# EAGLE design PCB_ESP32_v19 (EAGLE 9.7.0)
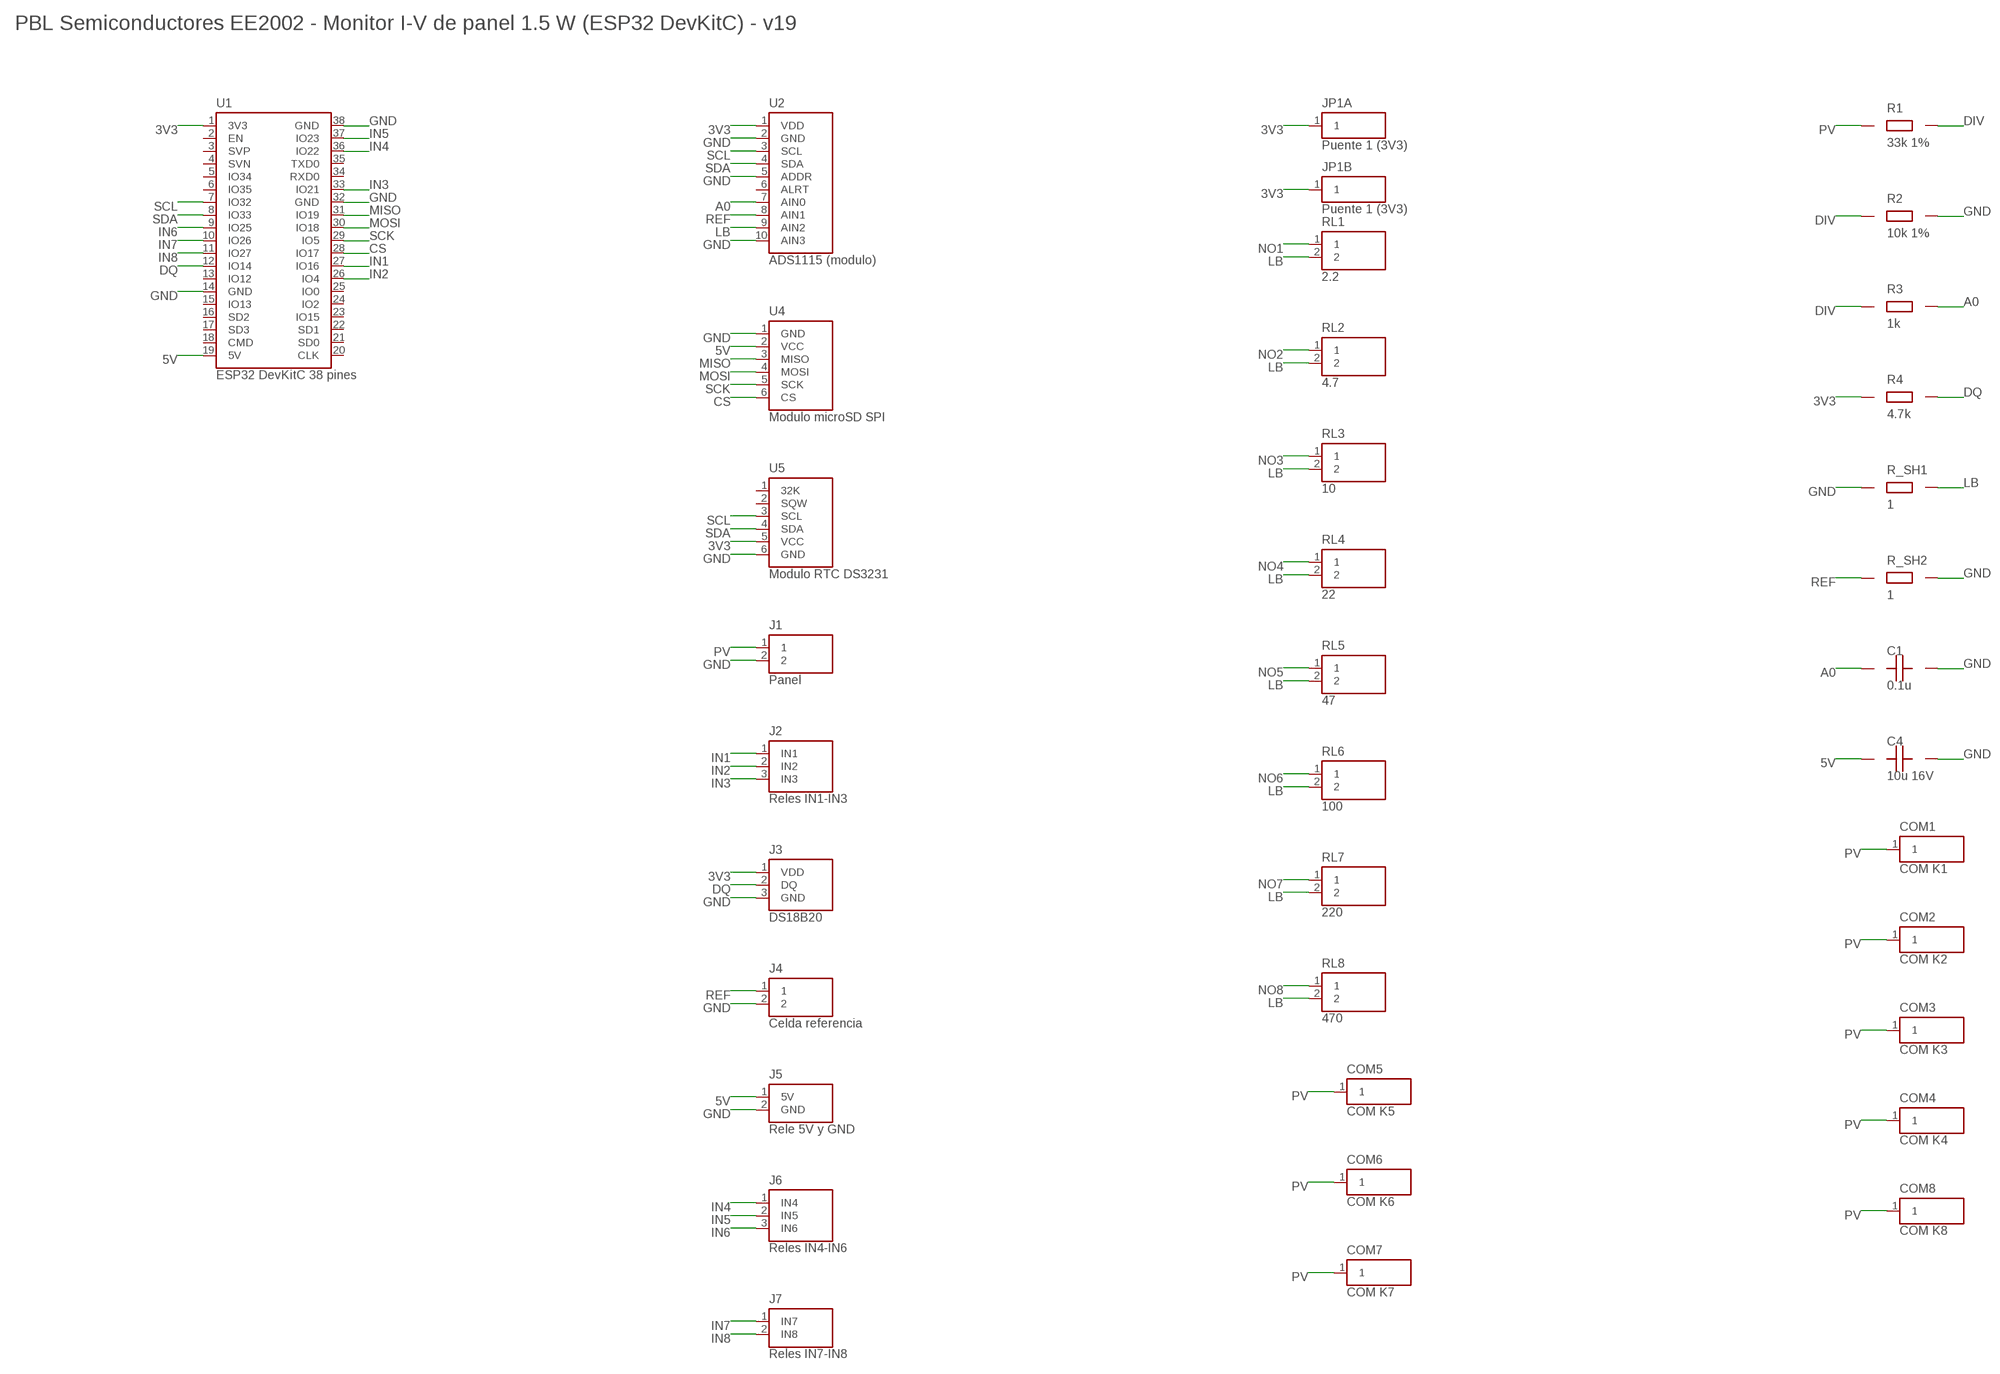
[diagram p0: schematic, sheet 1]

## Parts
C1  0.1u  C  [CAP_5MM]
C4  10u 16V  CP  [CAP_E_2_54]
COM1  COM K1  WIREPAD  [WIREPAD]
COM2  COM K2  WIREPAD  [WIREPAD]
COM3  COM K3  WIREPAD  [WIREPAD]
COM4  COM K4  WIREPAD  [WIREPAD]
COM5  COM K5  WIREPAD  [WIREPAD]
COM6  COM K6  WIREPAD  [WIREPAD]
COM7  COM K7  WIREPAD  [WIREPAD]
COM8  COM K8  WIREPAD  [WIREPAD]
J1  Panel  TERM2  [TERM2_5MM]
J2  Reles IN1-IN3  RELAY_L  [MALE_1X03]
J3  DS18B20  DS18B20_HDR  [MALE_1X03]
J4  Celda referencia  TERM2  [TERM2_5MM]
J5  Rele 5V y GND  RELAY_PWR  [MALE_1X02]
J6  Reles IN4-IN6  RELAY_RA  [MALE_1X03]
J7  Reles IN7-IN8  RELAY_RC  [MALE_1X02]
JP1A  Puente 1 (3V3)  JPAD  [JPAD]
JP1B  Puente 1 (3V3)  JPAD  [JPAD]
R1  33k 1%  R  [RES_V]
R2  10k 1%  R  [RES_V]
R3  1k  R  [RES_V]
R4  4.7k  R  [RES_V]
R_SH1  1  R  [RES_V]
R_SH2  1  R  [RES_V]
RL1  2.2  RLOAD  [RES_H_T]
RL2  4.7  RLOAD  [RES_H_T]
RL3  10  RLOAD  [RES_H_T]
RL4  22  RLOAD  [RES_H_T]
RL5  47  RLOAD  [RES_H_T]
RL6  100  RLOAD  [RES_H_T]
RL7  220  RLOAD  [RES_H_T]
RL8  470  RLOAD  [RES_H_T]
U1  ESP32 DevKitC 38 pines  ESP32  [ESP32_DEVKIT38]
U2  ADS1115 (modulo)  ADS1115  [SOCKET_1X10]
U4  Modulo microSD SPI  SDCARD  [SOCKET_1X06]
U5  Modulo RTC DS3231  DS3231  [SOCKET_1X06]

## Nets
3V3 [POWER]: J3.1(VDD) JP1A.1 JP1B.1 R4.1 U1.1(3V3) U2.1(VDD) U5.5(VCC)
5V [POWER]: C4.1(+) J5.1(5V) U1.19(5V) U4.2(VCC)
A0: C1.1 R3.2 U2.7(AIN0)
CS: U1.28(IO17) U4.6(CS)
DIV: R1.2 R2.1 R3.1
DQ: J3.2(DQ) R4.2 U1.12(IO14)
GND [POWER]: C1.2 C4.2(-) J1.2 J3.3(GND) J4.2 J5.2(GND) R2.2 R_SH1.1 R_SH2.2 U1.14(GND) U1.32(GND) U1.38(GND) U2.2(GND) U2.5(ADDR) U2.10(AIN3) U4.1(GND) U5.6(GND)
IN1: J2.1(IN1) U1.27(IO16)
IN2: J2.2(IN2) U1.26(IO4)
IN3: J2.3(IN3) U1.33(IO21)
IN4: J6.1(IN4) U1.36(IO22)
IN5: J6.2(IN5) U1.37(IO23)
IN6: J6.3(IN6) U1.9(IO25)
IN7: J7.1(IN7) U1.10(IO26)
IN8: J7.2(IN8) U1.11(IO27)
LB [POWER]: R_SH1.2 RL1.2 RL2.2 RL3.2 RL4.2 RL5.2 RL6.2 RL7.2 RL8.2 U2.9(AIN2)
MISO: U1.31(IO19) U4.3(MISO)
MOSI: U1.30(IO18) U4.4(MOSI)
NO1: RL1.1
NO2: RL2.1
NO3: RL3.1
NO4: RL4.1
NO5: RL5.1
NO6: RL6.1
NO7: RL7.1
NO8: RL8.1
PV [POWER]: COM1.1 COM2.1 COM3.1 COM4.1 COM5.1 COM6.1 COM7.1 COM8.1 J1.1 R1.1
REF: J4.1 R_SH2.1 U2.8(AIN1)
SCK: U1.29(IO5) U4.5(SCK)
SCL: U1.7(IO32) U2.3(SCL) U5.3(SCL)
SDA: U1.8(IO33) U2.4(SDA) U5.4(SDA)
Unconnected: U1.2(EN) U1.3(SVP) U1.4(SVN) U1.5(IO34) U1.6(IO35) U1.13(IO12) U1.15(IO13) U1.16(SD2) U1.17(SD3) U1.18(CMD) U1.20(CLK) U1.21(SD0) U1.22(SD1) U1.23(IO15) U1.24(IO2) U1.25(IO0) U1.34(RXD0) U1.35(TXD0) U2.6(ALRT) U5.1(32K) U5.2(SQW)

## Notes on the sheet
- PBL Semiconductores EE2002 - Monitor I-V de panel 1.5 W (ESP32 DevKitC) - v19

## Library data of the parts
C1 = PCB_PBL_Semiconductores:C
C4 = PCB_PBL_Semiconductores:CP
COM1-COM8 = PCB_PBL_Semiconductores:WIREPAD
J1 J4 = PCB_PBL_Semiconductores:TERM2
J2 = PCB_PBL_Semiconductores:RELAY_L
J3 = PCB_PBL_Semiconductores:DS18B20_HDR
J5 = PCB_PBL_Semiconductores:RELAY_PWR
J6 = PCB_PBL_Semiconductores:RELAY_RA
J7 = PCB_PBL_Semiconductores:RELAY_RC
JP1A JP1B = PCB_PBL_Semiconductores:JPAD
R1-R4 R_SH1 R_SH2 = PCB_PBL_Semiconductores:R
RL1-RL8 = PCB_PBL_Semiconductores:RLOAD
U1 = PCB_PBL_Semiconductores:ESP32
U2 = PCB_PBL_Semiconductores:ADS1115
U4 = PCB_PBL_Semiconductores:SDCARD
U5 = PCB_PBL_Semiconductores:DS3231

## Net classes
0 SIGNAL: width 0.254 mm, drill 0.381 mm, clearance 0.254 mm
1 POWER: width 0.381 mm, drill 0.508 mm, clearance 0.305 mm to class 0, clearance 0.305 mm

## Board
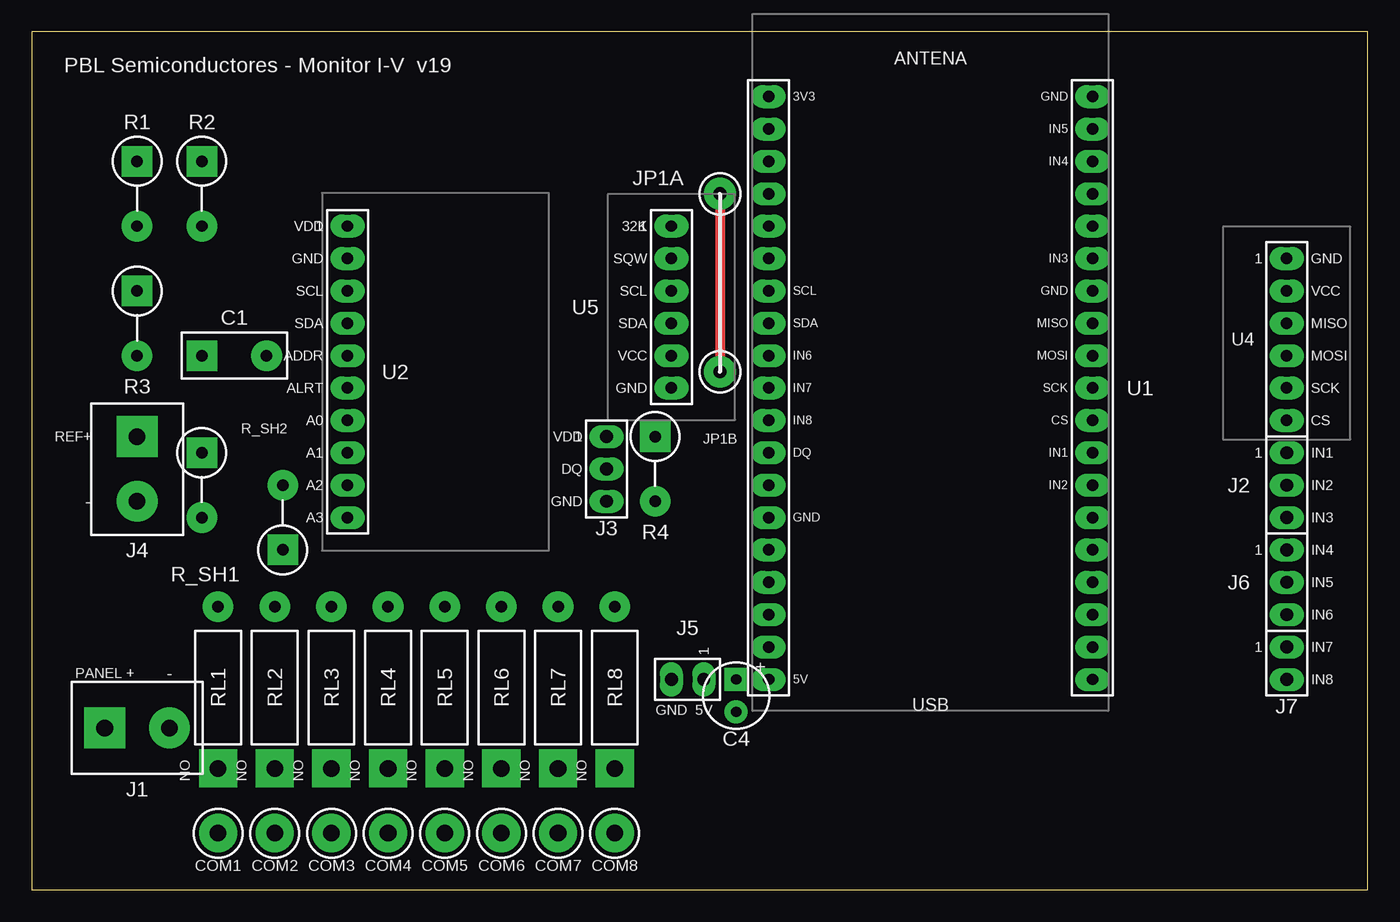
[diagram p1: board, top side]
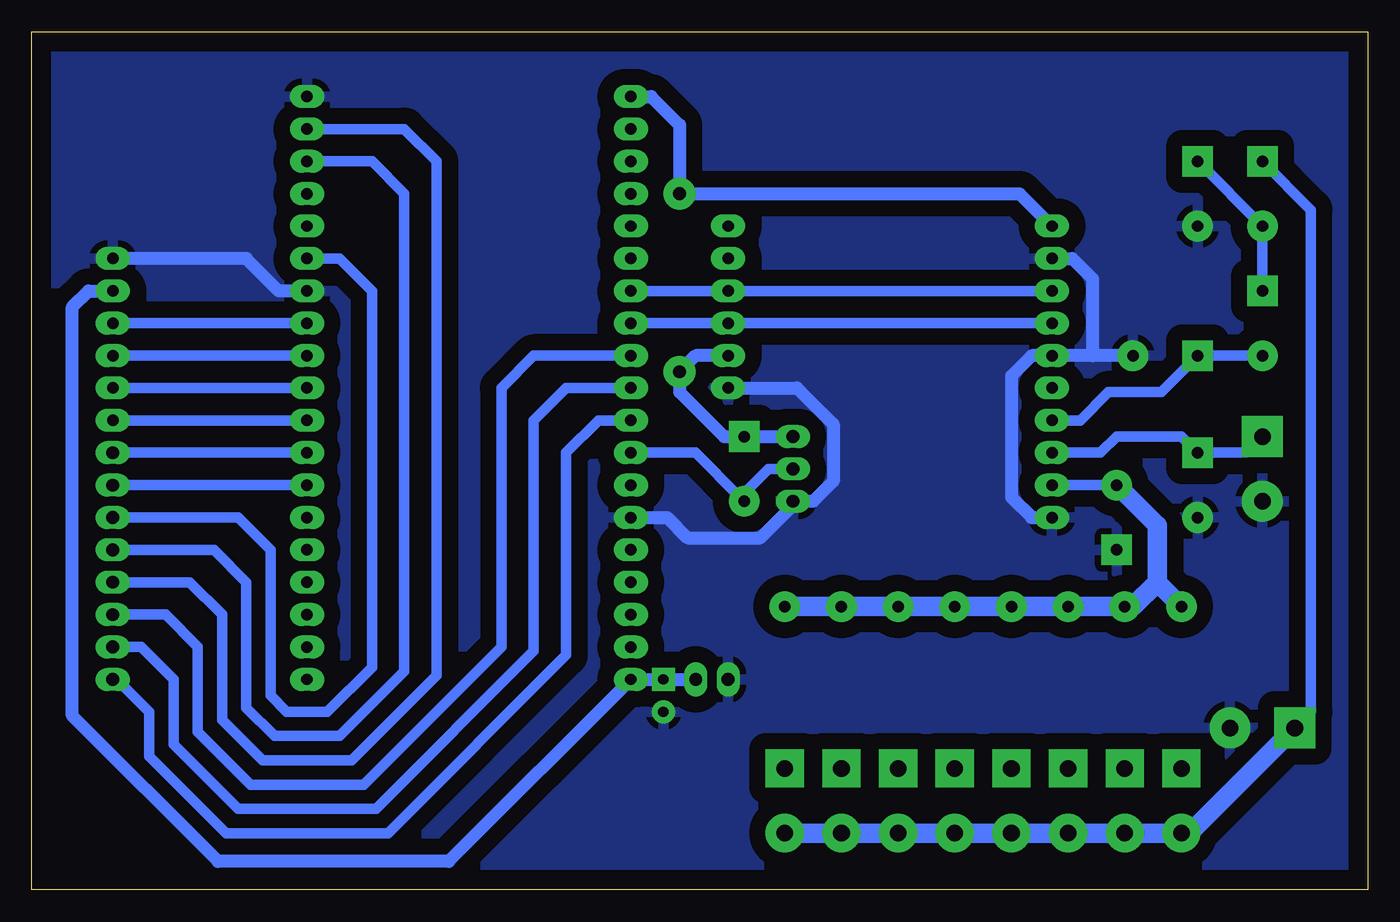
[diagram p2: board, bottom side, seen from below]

Size 104.78 x 67.31 mm. Coordinates in mm from the lower left corner, seen from the top.
Outline: 0,0 104.78,0 104.78,67.31 0,67.31 0,0
Copper layers (1*16): Top 0.035mm / dielectric 1.5mm / Bottom 0.035mm
Design rules "PBL v19 (mil, planchado / percloruro)": minimum track width 10mil, minimum drill 15mil, track to track 40mil, track to pad 40mil, pad to pad 20mil, via to via 20mil, smd to smd 6mil, copper to edge 60mil, drill to drill 6mil, minimum pad ring 0.4mm, minimum via ring 0.4mm, stop-mask expansion 4mil, vias tented up to drill 9999mil, thermal gap 20mil

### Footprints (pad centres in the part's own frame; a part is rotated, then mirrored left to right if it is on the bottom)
CAP_5MM = drill 0.9 pad 2.4 square: 1 0,0 | drill 0.9 pad 2.4 round: 2 5.08,0
CAP_E_2_54 = drill 0.8 pad 1.8 square: 1 0,0 | drill 0.8 pad 1.8 round: 2 2.54,0
WIREPAD = drill 1.3 pad 3 round: 1 0,0
TERM2_5MM = drill 1.3 pad 3.2 square: 1 0,0 | drill 1.3 pad 3.2 round: 2 5.08,0
MALE_1X03 = drill 1 pad 1.8 long: 1 0,0; 2 0,-2.54; 3 0,-5.08
MALE_1X02 = drill 1 pad 1.8 long: 1 0,0; 2 0,-2.54
JPAD = drill 1 pad 2.5 round: 1 0,0
RES_V = drill 0.9 pad 2.4 square: 1 0,0 | drill 0.9 pad 2.4 round: 2 5.08,0
RES_H_T = drill 1.3 pad 3 square: 1 0,0 | drill 0.9 pad 2.4 round: 2 12.7,0
ESP32_DEVKIT38 = drill 0.9 pad 1.8 long: 1 0,0; 2 0,-2.54; 3 0,-5.08; 4 0,-7.62; 5 0,-10.16; 6 0,-12.7; 7 0,-15.24; 8 0,-17.78; 9 0,-20.32; 10 0,-22.86; 11 0,-25.4; 12 0,-27.94; 13 0,-30.48; 14 0,-33.02; 15 0,-35.56; 16 0,-38.1; 17 0,-40.64; 18 0,-43.18; 19 0,-45.72; 20 25.4,-45.72; 21 25.4,-43.18; 22 25.4,-40.64; 23 25.4,-38.1; 24 25.4,-35.56; 25 25.4,-33.02; 26 25.4,-30.48; 27 25.4,-27.94; 28 25.4,-25.4; 29 25.4,-22.86; 30 25.4,-20.32; 31 25.4,-17.78; 32 25.4,-15.24; 33 25.4,-12.7; 34 25.4,-10.16; 35 25.4,-7.62; 36 25.4,-5.08; 37 25.4,-2.54; 38 25.4,0
SOCKET_1X10 = drill 0.9 pad 1.8 long: 1 0,0; 2 0,-2.54; 3 0,-5.08; 4 0,-7.62; 5 0,-10.16; 6 0,-12.7; 7 0,-15.24; 8 0,-17.78; 9 0,-20.32; 10 0,-22.86
SOCKET_1X06 = drill 0.9 pad 1.8 long: 1 0,0; 2 0,-2.54; 3 0,-5.08; 4 0,-7.62; 5 0,-10.16; 6 0,-12.7

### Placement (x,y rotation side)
C1  13.34,41.91 0 top
C4  55.24,16.51 270 top
COM1  14.61,4.45 0 top
COM2  19.05,4.45 0 top
COM3  23.5,4.45 0 top
COM4  27.94,4.45 0 top
COM5  32.38,4.45 0 top
COM6  36.83,4.45 0 top
COM7  41.27,4.45 0 top
COM8  45.72,4.45 0 top
J1  5.71,12.7 0 top
J2  98.42,34.29 0 top
J3  45.09,35.56 0 top
J4  8.26,35.56 270 top
J5  52.7,16.51 270 top
J6  98.42,26.67 0 top
J7  98.42,19.05 0 top
JP1A  53.98,54.61 0 top
JP1B  53.98,40.64 0 top
R1  8.26,57.15 270 top
R2  13.34,57.15 270 top
R3  8.26,46.99 270 top
R4  48.9,35.56 270 top
R_SH1  19.68,26.67 90 top
R_SH2  13.34,34.29 270 top
RL1  14.61,9.53 90 top
RL2  19.05,9.53 90 top
RL3  23.5,9.53 90 top
RL4  27.94,9.53 90 top
RL5  32.38,9.53 90 top
RL6  36.83,9.53 90 top
RL7  41.27,9.53 90 top
RL8  45.72,9.53 90 top
U1  57.78,62.23 0 top
U2  24.77,52.07 0 top
U4  98.42,49.53 0 top
U5  50.16,52.07 0 top

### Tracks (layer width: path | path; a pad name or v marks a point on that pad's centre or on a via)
3V3
  Top 0.8: JP1A.1 JP1B.1
  Bottom 1.016: U1.1 56.2,62.23 53.98,60.01 JP1A.1 27.3,54.61 U2.1 | U5.5 52.7,41.91 JP1B.1 53.98,39.05 50.48,35.56 R4.1 J3.1
5V
  Bottom 1.016: J5.1 C4.1 U1.19 72.07,2.22 90.17,2.22 101.6,13.65 101.6,45.72 100.33,46.99 U4.2
A0
  Bottom 0.813: U2.7 22.54,36.83 20.32,39.05 16.19,39.05 C1.1 R3.2
CS
  Bottom 0.813: U1.28 U4.6
DIV
  Bottom 0.813: R3.1 R1.2 R2.1
DQ
  Bottom 0.813: U1.12 52.7,34.29 49.21,30.8 | 49.21,30.8 R4.2 | 49.21,30.8 46.99,33.02 J3.2
GND
  Bottom 1.016: C1.2 21.59,41.91 | 21.59,41.91 U2.5 26.35,41.91 27.94,40.32 27.94,30.8 26.35,29.21 U2.10 | U2.2 23.18,49.53 21.59,47.94 21.59,41.91 | U1.14 54.93,29.21 53.34,27.62 47.62,27.62 45.09,30.16 J3.3 43.5,30.48 41.91,32.07 41.91,36.51 44.77,39.37 U5.6 | U1.32 85.41,46.99 87.95,49.53 U4.1
  pour Bottom (isolate 1.27): 0.5,0.5 104.28,0.5 104.28,66.81 0.5,66.81
IN1
  Bottom 0.813: U1.27 J2.1
IN2
  Bottom 0.813: U1.26 J2.2
IN3
  Bottom 0.813: U1.33 80.64,49.53 78.11,46.99 78.11,17.46 81.6,13.97 84.77,13.97 86.04,15.24 86.04,26.67 88.58,29.21 J2.3
IN4
  Bottom 0.813: U1.36 78.11,57.15 75.56,54.61 75.56,17.14 80.64,12.06 85.72,12.06 87.95,14.29 87.95,24.13 90.49,26.67 J6.1
IN5
  Bottom 0.813: U1.37 75.56,59.69 73.03,57.15 73.03,16.83 79.69,10.16 86.68,10.16 89.85,13.34 89.85,21.59 92.39,24.13 J6.2
IN6
  Bottom 0.813: U1.9 65.41,41.91 67.94,39.37 67.94,19.05 78.74,8.26 87.63,8.26 91.76,12.38 91.76,19.05 94.3,21.59 J6.3
IN7
  Bottom 0.813: U1.10 62.87,39.37 65.41,36.83 65.41,18.73 77.79,6.35 88.58,6.35 93.66,11.43 93.66,16.51 96.2,19.05 J7.1
IN8
  Bottom 0.813: U1.11 60.33,36.83 62.87,34.29 62.87,18.41 76.83,4.45 89.53,4.45 95.57,10.48 95.57,13.97 98.11,16.51 J7.2
LB
  Bottom 0.813: U2.9 R_SH1.2
  Bottom 1.524: R_SH1.2 16.51,28.57 16.51,24.13 | 16.51,24.13 RL1.2 | 16.51,24.13 18.41,22.23 RL2.2 RL3.2 RL4.2 RL5.2 RL6.2 RL7.2 RL8.2
MISO
  Bottom 0.813: U1.31 U4.3
MOSI
  Bottom 0.813: U1.30 U4.4
PV
  Bottom 0.813: J1.1 4.45,13.97 4.45,53.34 R1.1
  Bottom 1.524: J1.1 13.97,4.45 COM1.1 COM2.1 COM3.1 COM4.1 COM5.1 COM6.1 COM7.1 COM8.1
REF
  Bottom 0.813: U2.8 20.95,34.29 19.68,35.56 14.61,35.56 R_SH2.1 9.53,34.29 J4.1
SCK
  Bottom 0.813: U1.29 U4.5
SCL
  Bottom 0.813: U1.7 U5.3 U2.3
SDA
  Bottom 0.813: U1.8 U5.4 U2.4

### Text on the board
tPlace: PBL Semiconductores - Monitor I-V v19 | 3V3 | GND | IN5 | IN4 | VDD | 32K | GND | SQW | IN3 | GND | SCL | SCL | SCL | GND | VCC | SDA | SDA | SDA | MISO | MISO | ADDR | VCC | IN6 | MOSI | MOSI | ALRT | GND | IN7 | SCK | SCK | A0 | IN8 | CS | CS | REF+ | VDD | A1 | DQ | IN1 | IN1 | DQ | A2 | IN2 | IN2 | - | GND | A3 | GND | IN3 | IN4 | IN5 | IN6 | IN7 | PANEL + | - | 5V | IN8 | GND | 5V
tDocu: ADS1115 (modulo plano, 28x17.8) | RTC parado (pines en L) | microSD parada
